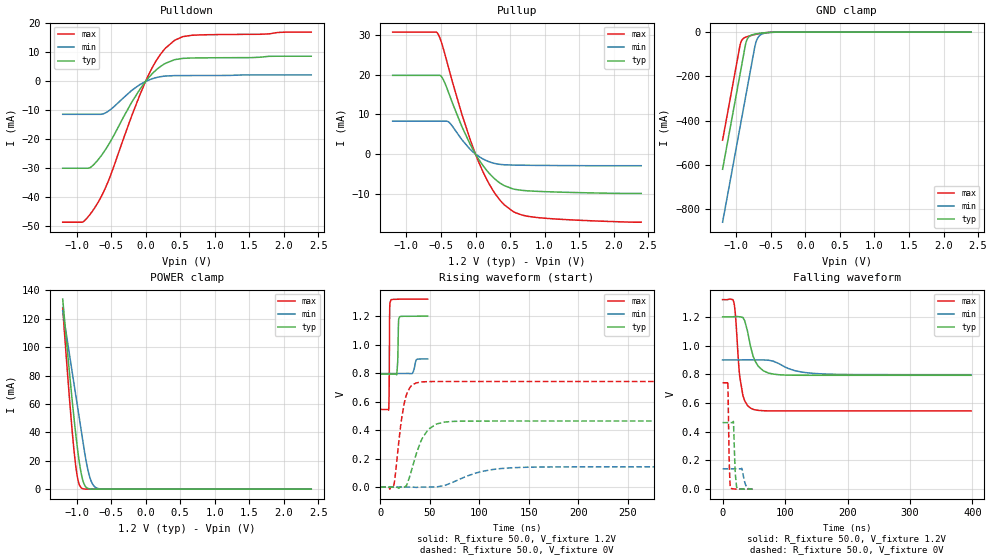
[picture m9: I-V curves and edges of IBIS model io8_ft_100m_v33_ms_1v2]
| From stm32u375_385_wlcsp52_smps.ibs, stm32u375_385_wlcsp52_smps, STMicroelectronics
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[Model]   io8_ft_100m_v33_ms_1v2
Model_type I/O
Polarity   Non-Inverting
Enable   Active-Low
| CAP_THRESHOLD on pad IOFT is "UDTCAPC" :
| Rising=30.0% of vddiom   Falling=70.0% of vddiom
| C_comp min and max val. don't necessarily correlate with the min and max pvt
| but are the smallest and greatest pad capacitance found.
| var   typ   min   max
C_comp   3.62609pF  3.42535pF  3.70436pF
|C_comp_pullup   2.21485pF  1.92182pF  2.35475pF
|C_comp_pulldown   1.41124pF  1.50353pF  1.34960pF
Vinl = 450.0mV
Vinh = 660.0mV
Vmeas = 600.0mV   | Reference voltage for timing measurements
Cref  = 50.0pF   | Timing specification test load capacitance value
Rref  = 1.0MOhm   | Timing specification test load resistance value
Vref  = 660.0mV   | Timing specification test load voltage
[Model Spec]
| TIME_THRESHOLD on pin ZIV33M is "CMOS" :
| Rising=50.0% of vddiom   Falling=50.0% of vddiom
Vinl 434.50000mV 327.50000mV 480.50000mV
Vinh 750.50000mV 549.50000mV 835.50000mV
| variable   typ   min   max
[Temperature Range] 25.0 130.0 -40.0
| variable   typ   min   max
[Voltage Range] 1.2V 900.0mV 1.32V
| variable   typ   min   max
[POWER Clamp Reference] 1.2V 900.0mV 1.32V
| variable   typ   min   max
[GND Clamp Reference] 0V 0V 0V
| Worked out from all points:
|   slope of the pulldown table from 0 to 0.18 V, typ, clamps not added: 40 ohm
|   slope of the pullup table from 0 to 0.18 V, typ, clamps not added: 40 ohm
|   GND clamp passes 1 mA (typ) near -0.50 V on its own axis
|   POWER clamp passes 1 mA (typ) near -0.85 V on its own axis
|   rising waveform, R_fixture 50.0, V_fixture 1.2V: 20-80 % time 753ps typ, 1.98ns min, 398ps max; typ from 0.793 V to 1.2 V
|   falling waveform, R_fixture 50.0, V_fixture 1.2V: 20-80 % time 15.8ns typ, 36.5ns min, 9.29ns max; typ from 1.2 V to 0.793 V
|   rising waveform, R_fixture 50.0, V_fixture 0V: 20-80 % time 14.6ns typ, 34ns min, 8.15ns max; typ from 0 V to 0.464 V
|   falling waveform, R_fixture 50.0, V_fixture 0V: 20-80 % time 2.51ns typ, 4.64ns min, 1.89ns max; typ from 0.464 V to 0 V
[POWER Clamp]
-1.2V     133.8mA    125.6mA    127.5mA
-1.08V    70.97mA    87.88mA    50.75mA
-1.04V    51.73mA    75.31mA    29.13mA
-1.01V    38.33mA    65.88mA    15.91mA
-970mV    22.56mA    53.3mA     4.74mA
-930mV    10.55mA    40.73mA    892.2uA
-890mV    3.611mA    28.15mA    138.3uA
-850mV    950.4uA    17.03mA    20.6uA
-810mV    222.1uA    8.794mA    3.05uA
-770mV    50.16uA    3.803mA    451.1nA
-650mV    561.7nA    165.6uA    1.537nA
2.4V      0A         0A         0A
[GND Clamp]
-1.2V     -620mA     -859.4mA   -488.5mA
-940mV    -178mA     -417.4mA   -50.52mA
-910mV    -127mA     -366.4mA   -31.92mA
-870mV    -59.03mA   -298.4mA   -23.56mA
-840mV    -30.06mA   -247.4mA   -20.12mA
-800mV    -16.5mA    -179.4mA   -16.42mA
-730mV    -9.175mA   -61.6mA    -10.9mA
-700mV    -7.461mA   -32.04mA   -8.862mA
-660mV    -5.584mA   -14.78mA   -6.456mA
-570mV    -2.482mA   -3.888mA   -2.491mA
-380mV    -62.94uA   -244.6uA   -21.21uA
2.4V      891.3pA    142.1nA    382.4pA
| variable   typ   min   max
[Pullup Reference] 1.2V 900.0mV 1.32V
| variable   typ   min   max
[Pulldown Reference] 0V 0V 0V
[Pullup]
-1.2V     19.88mA    8.293mA    30.81mA
-550mV    19.88mA    8.293mA    30.54mA
-480mV    19.23mA    8.293mA    27.47mA
-380mV    15.05mA    7.965mA    21.15mA
-200mV    7.047mA    3.684mA    10.21mA
10mV      -293.8uA   -130.6uA   -448.5uA
210mV     -5.089mA   -2.027mA   -7.926mA
310mV     -6.737mA   -2.489mA   -10.64mA
420mV     -8mA       -2.709mA   -12.87mA
580mV     -8.947mA   -2.8mA     -14.83mA
790mV     -9.331mA   -2.845mA   -15.82mA
2.4V      -9.943mA   -2.948mA   -17.22mA
[Pulldown]
-1.2V     -29.93mA   -11.33mA   -48.55mA
-910mV    -29.93mA   -11.33mA   -48.48mA
-810mV    -29.8mA    -11.33mA   -46.03mA
-710mV    -27.65mA   -11.33mA   -42.6mA
-620mV    -24.89mA   -11.22mA   -38.69mA
-530mV    -21.58mA   -10.08mA   -33.79mA
-200mV    -7.157mA   -3.075mA   -11.82mA
40mV      1.18mA     424.7uA    2.081mA
230mV     5.395mA    1.701mA    9.799mA
420mV     7.512mA    2.016mA    14.19mA
670mV     8.097mA    2.046mA    15.93mA
2.4V      8.706mA    2.25mA     17.03mA
[Ramp]
dV/dt_r 278.13962mV/14.18091ns 85.18433mV/33.85286ns 444.65518mV/8.14507ns
dV/dt_f 244.21059mV/15.21254ns 61.56262mV/35.99177ns 465.10836mV/8.71121ns
R_load = 50.0
| Removed startup time: 0s 0s 0s  .
| Removed end time: 47.95ns.
[Rising Waveform]
R_fixture   = 50.0
V_fixture   = 1.2V
V_fixture_min = 900.0mV
V_fixture_max = 1.32V
0s        793mV      797.4mV    544.8mV
8.55ns    793mV      797.4mV    543mV
9.05ns    793mV      797.4mV    703.1mV
9.6ns     793mV      797.4mV    1.257V
10.8ns    793mV      797.4mV    1.315V
16.75ns   788.4mV    797.4mV    1.319V
17.65ns   882.1mV    797.4mV    1.319V
18.55ns   1.167V     797.4mV    1.319V
19.6ns    1.196V     797.4mV    1.319V
47.95ns   1.2V       899.6mV    1.32V
| Removed startup time: 0s 0s 0s  .
| Removed end time: 397.95ns.
[Falling Waveform]
R_fixture   = 50.0
V_fixture   = 1.2V
V_fixture_min = 900.0mV
V_fixture_max = 1.32V
0s        1.2V       900mV      1.32V
18ns      1.201V     900mV      1.301V
20.7ns    1.201V     900mV      1.205V
27.2ns    1.2V       900mV      795.7mV
32.5ns    1.196V     900.6mV    652.9mV
48.75ns   927.5mV    900.5mV    556.6mV
65ns      824.9mV    899.9mV    546.3mV
89.35ns   797.2mV    876.1mV    544.9mV
154.4ns   793mV      803.9mV    544.8mV
398ns     793mV      797.4mV    544.8mV
| Removed startup time: 0s 0s 0s  .
| Removed end time: 397.9ns.
[Rising Waveform]
R_fixture   = 50.0
V_fixture   = 0V
V_fixture_min = 0V
V_fixture_max = 0V
0s        4.987nV    173.7nV    3.506nV
13.45ns   2.494uV    172.6nV    7.951mV
20.6ns    -669uV     627.5nV    427.5mV
24.35ns   718uV      991.1nV    591.5mV
30ns      78.47mV    46.1uV     699.4mV
36.55ns   236.1mV    -2.258mV   731.4mV
48.75ns   406.4mV    89.58uV    740.3mV
64.95ns   456.2mV    10.71mV    741mV
129.9ns   463.5mV    134.2mV    741.1mV
397.9ns   463.6mV    142mV      741.1mV
| Removed startup time: 0s 0s 0s  .
| Removed end time: 47.95ns.
[Falling Waveform]
R_fixture   = 50.0
V_fixture   = 0V
V_fixture_min = 0V
V_fixture_max = 0V
0s        463.6mV    142mV      741.1mV
8.35ns    463.6mV    142mV      749.2mV
10.65ns   463.6mV    142mV      190.8mV
12.75ns   463.6mV    142mV      9.005mV
17.35ns   469.6mV    142mV      2.186mV
20.3ns    116.9mV    142mV      1.037mV
22.55ns   13.65mV    142mV      577.5uV
30.65ns   873.3uV    145.6mV    137.5uV
37.2ns    463uV      26.99mV    56.59uV
47.95ns   183.8uV    1.322mV    13.5uV
